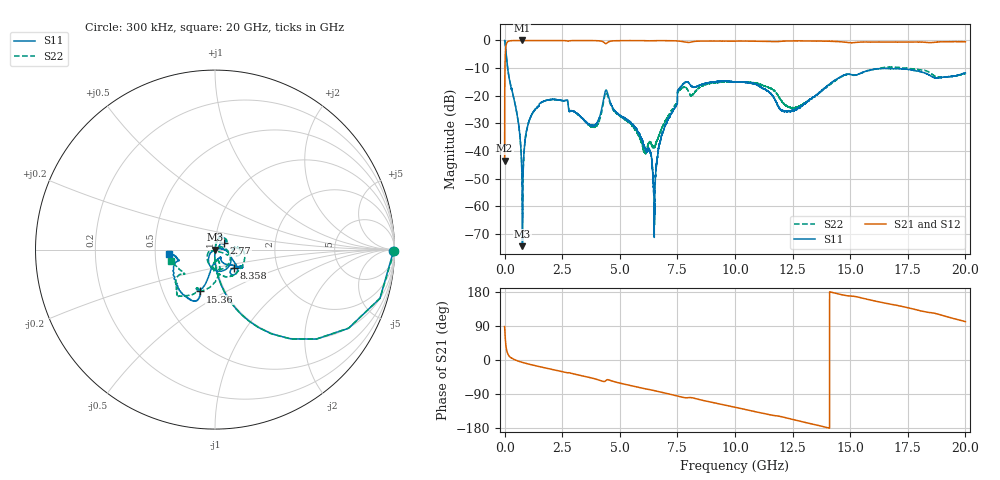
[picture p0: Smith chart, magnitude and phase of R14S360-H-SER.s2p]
!{R14S360}
!Johanson Technology Inc.
!www.johansontechnology.com
!Test Board Conditions:
!Substrate Type  RO4350B
!Substrate Thickness  20 mil
!Substrate Dk  3.66
!TL Type: GCPW
!TL Trace Width  36 mil
!TL Gap  12 mil
!Electrode orientation  Horizontal
!DUT TOPOLOGY	SERIES
!Mounting Pad LxW  26x36 mil
! Created Wed Nov 25 17:33:21 2020
! 2 Port Network Data from SP1.SP block
! freq  magS11  angS11  magS21  angS21  magS12  angS12  magS22  angS22
# khz S ma R 50
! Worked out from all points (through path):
!   20001 points, 300 kHz to 20 GHz, reference 50 ohm
!   highest |S21| = 0.00 dB at 760.3 MHz (marker M1); lowest = -43.5 dB at 300 kHz (marker M2)
!   group delay of S21, straight-line fit = 36.1 ps
!   lowest |S11| = -74.4 dB at 775.3 MHz (marker M3), VSWR 1.00, Z = 50 + j0.0158 ohm
!   |S11| at or under -10 dB: 131.9 MHz to end of sweep
!   |S22| runs from -64.1 to 0.0 dB; largest |S21 - S12| = 0.019
!   S11 on the Smith chart (normalised r, x): 300 kHz: open; 2.77 GHz: 1.10, +0.08; 8.358 GHz: 1.21, -0.26; 15.36 GHz: 0.76, -0.38; 20 GHz: 0.59, -0.03
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300  0.9941 -0.6  0.00666 88.3  0.006516 89.6  0.9985 -0.5
124300  0.3339 -71.5  0.9409 18.4  0.9417 18.5  0.3353 -71.4
566300  0.03972 -92.0  0.9987 -2.2  0.9989 -2.3  0.04 -91.9
760300  0.002671 -98.3  0.9999 -6.1  0.9983 -6.0  0.003163 -84.3
775300  0.0001898 123.6  0.9987 -6.4  0.9997 -6.3  0.000868 -44.7
993300  0.02783 80.4  0.9981 -10.0  0.9993 -10.0  0.02769 78.0
1302300  0.055 76.2  0.9977 -14.5  0.997 -14.5  0.05497 73.9
2770300  0.06134 35.4  0.97 -33.5  0.9705 -33.4  0.06571 29.2
3334300  0.04039 47.0  0.9957 -41.3  0.9964 -41.3  0.03994 45.4
3962300  0.03012 18.8  0.9914 -50.4  0.9908 -50.4  0.02774 37.2
4423300  0.1251 -75.9  0.8858 -52.9  0.8852 -52.9  0.1143 -75.5
6289300  0.01031 -117.7  0.9842 -78.2  0.9851 -78.2  0.01416 -90.6
6489300  0.001128 -152.1  0.9914 -80.7  0.9911 -80.7  0.01209 -70.1
6667300  0.0103 16.5  0.9922 -83.2  0.9914 -83.2  0.01778 -36.3
7600300  0.1381 -34.3  0.97 -96.6  0.97 -96.5  0.1271 5.4
8358300  0.1486 -44.0  0.9686 -102.9  0.9679 -102.9  0.1302 4.7
1.00003e7  0.1787 -30.9  0.9725 -124.7  0.9722 -124.7  0.1763 -43.3
1.20943e7  0.05287 -54.1  0.9713 -150.7  0.9737 -150.7  0.07395 -95.3
1.33343e7  0.08893 -98.6  0.9767 -168.8  0.9786 -168.8  0.08862 -73.8
1.53643e7  0.2475 -109.8  0.9317 165.6  0.9358 165.4  0.2473 -113.3
1.66673e7  0.3093 -117.1  0.9378 148.3  0.9282 148.1  0.3312 -128.1
2e7  0.2586 -174.9  0.9467 101.2  0.9465 101.4  0.2519 -165.2
